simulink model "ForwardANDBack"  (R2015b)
settings: Solver=FixedStepDiscrete  StartTime=0.0  StopTime=10.0  RelTol=1e-3
libraries: vexarmcortexlib x4

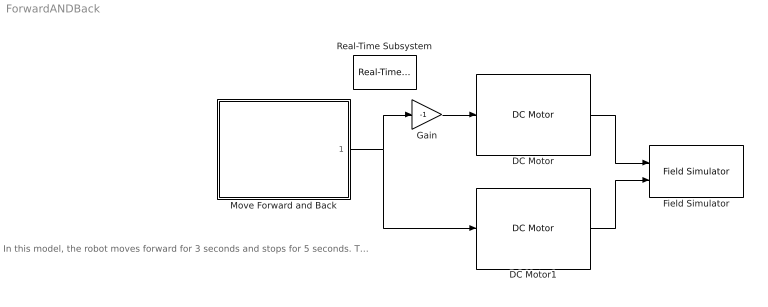
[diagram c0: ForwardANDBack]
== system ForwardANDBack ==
  note: In this model, the robot moves forward for 3 seconds and stops for 5 seconds. Then the robot will move in reverse for 7 seconds.
  DC Motor : vexarmcortexlib/DC Motor  motor=3  scaleFactor=1/13.5  SimulationOut=on
  DC Motor1 : vexarmcortexlib/DC Motor  motor=7  scaleFactor=1/13.5  SimulationOut=on
  Field Simulator : vexarmcortexlib/Utilities/Field Simulator  radius=2.5  space=10  range=200
  Gain : Gain  Gain=-1
  Move Forward and Back : Stateflow chart  TreatAsAtomicUnit=on
  Real-Time Subsystem : vexarmcortexlib/Utilities/Real-Time Subsystem  x=1
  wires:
  Gain/1 -> DC Motor/1
  DC Motor/1 -> Field Simulator/1
  DC Motor1/1 -> Field Simulator/2
  Move Forward and Back/1(speed1) -> Gain/1, DC Motor1/1

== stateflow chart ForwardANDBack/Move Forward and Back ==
  state Drive_Forward
    during:
    speed1 = 100;
  state Halt
    during:
    speed1 = 0;
  state Drive_Backward
    during:
    speed1 = -100;
  state Stop
    during:
    speed1 = 0;
  (default) -> Drive_Forward : {speed1 = 0;}
  Drive_Forward -> Halt : after(2,sec)
  Halt -> Drive_Backward : after(3,sec)
  Drive_Backward -> Stop : after(5,sec)
  data: speed1 output
